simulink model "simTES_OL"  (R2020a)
settings: Solver=ode15s  StartTime=0.0  StopTime=tsim  RelTol=1e-3
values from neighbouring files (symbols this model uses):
  d0 = [qS0;qnom]    [runTES.m]    (also in Main.m = [Fh, Tcin, Thin]; Main_OL.m = [Fh, Tcin, Thin]; runTestCalcBlk.m = [Fh, Tcin, Thin]; runTransf.m = [Fh; Tcin; U0; Ffeed0; m0; Tfeed0])
  df = [qS0;qnom*1.5]    [runTES.m]
  nd = length(d0)    [runTES.m]    (also in Main.m = size(d0,2); Main_OL.m = size(d0,2); runTestCalcBlk.m = size(d0,2); runTransf.m = size(d0,1))
  np = length(param)    [runTES.m]    (also in runH2Psim.m; Main.m = size(p,2); Main_OL.m = size(p,2); runTestCalcBlk.m = size(p,2))
  nu = length(u0)    [runTES.m]    (also in runH2Psim.m; Main.m = 1; Main_OL.m = 1; runTestCalcBlk.m = 1)
  nx = length(x0)    [runTES.m]    (also in H2P_Turbine_driven.m = param(end); runTD.m; H2P_Boiler_driven.m = param(end); runBD.m)
  param = [V;rho;p0;m0;eps;]    [runTES.m]    (also in runTD.m = [Tref;TrefB;dHvap;cpg;cpW;cpSt;R;Mwt;     T0;TG0;ME;pC;     ; runBD.m = [Tref;TrefB;dHvap;cpg;cpW;cpSt;R;Mwt;          T0;TG0;ME;pC;; runFP.m = [Tref;TrefB;dHvap;cpg;cpW;cpSt;R;Mwt;          T0;TG0;ME;pC;; runFPV2.m = [Tref;TrefB;dHvap;cpg;cpW;cpSt;R;Mwt;          T0;TG0;ME;pC;)
  tdstep = 2/3600    (= 0.000555555555556)    [runTES.m]
  tustep = 2/3600    (= 0.000555555555556)    [runTES.m]
  u0 = [qSP0; qTP0; qEB0]    [runTES.m]    (also in runH2Psim.m = [mG0;zV0;mP0;mB0;mA0]; calcblock.m = p(2); testfun.m = 5; u_function.m = 5)
  uf = [qSP0;qTP0+0; qEB0+0]    [runTES.m]
  x0 = [Vh0;p0]    [runTES.m]    (also in runTD.m = [TE0;TD0;TSh0;MD0; MSh0;w0;TA0;0;0;0;0;0;0;0;0;0]; runBD.m = [TE0;TD0;TSh0;MD0; MSh0;w0;TA0;0;0;0;0;0;0;0;0;0]; runFP.m = [TE0;TD0;TSh0;MD0; MSh0;w0;TA0;0;0;0;0;0;0;0]; runFPV2.m = [TE0;TD0;TSh0;MD0; MSh0;w0;TA0;0;0;0;0;0;0;0])
undefined symbols (not defined in the file or in its folder): TESmodel

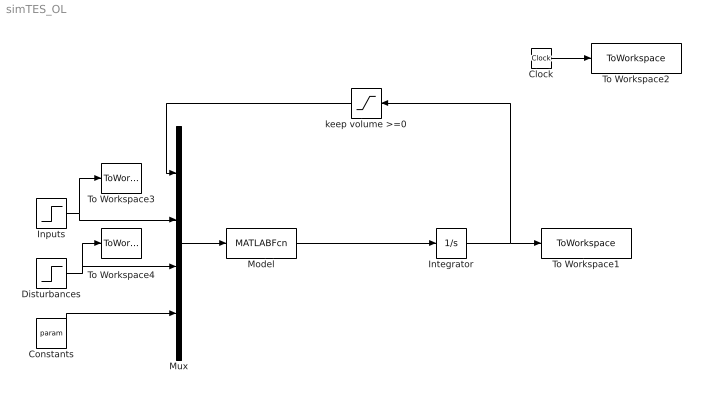
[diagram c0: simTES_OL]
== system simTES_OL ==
  Clock : Clock
  Constants : Constant  Value=param
  Disturbances : Step  Time=tdstep  Before=d0  After=df  SampleTime=0
  Inputs : Step  Time=tustep  Before=u0  After=uf  SampleTime=0
  Integrator : Integrator  InitialCondition=x0
  Model : MATLABFcn  MATLABFcn=TESmodel(u(1:nx),u(nx+1:nx+nu),u(nx+nu+1:nx+nu+nd),u(nx+nu+nd+1:nx+nu+nd+np))  OutputDimensions=nx
  Mux : Mux
  To Workspace1 : ToWorkspace  VariableName=yOL  SampleTime=-1
  To Workspace2 : ToWorkspace  VariableName=tOL  SampleTime=-1
  To Workspace3 : ToWorkspace  VariableName=uOL  SampleTime=-1
  To Workspace4 : ToWorkspace  VariableName=dOL  SampleTime=-1
  keep volume >=0 : Saturate  UpperLimit=inf  LowerLimit=0
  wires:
  Integrator/1 -> To Workspace1/1, keep volume >=0/1
  Mux/1 -> Model/1
  Constants/1 -> Mux/4
  Clock/1 -> To Workspace2/1
  keep volume >=0/1 -> Mux/1
  Disturbances/1 -> To Workspace4/1, Mux/3
  Inputs/1 -> To Workspace3/1, Mux/2
  Model/1 -> Integrator/1
